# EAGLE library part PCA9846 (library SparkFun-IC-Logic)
NXP Semiconductors PCA9846 - I2C Multiplexer The PCA9846 device has four bidirectional translating switches that can be controlled through the I2C bus. The SCL/SDA upstream pair fans out to four downstream pairs, or channels. Any individual SCn/SDn channel or combination of channels can be selected, determined by the contents of the programmable control register. These downstream channels can be used to resolve I2C address conflicts.
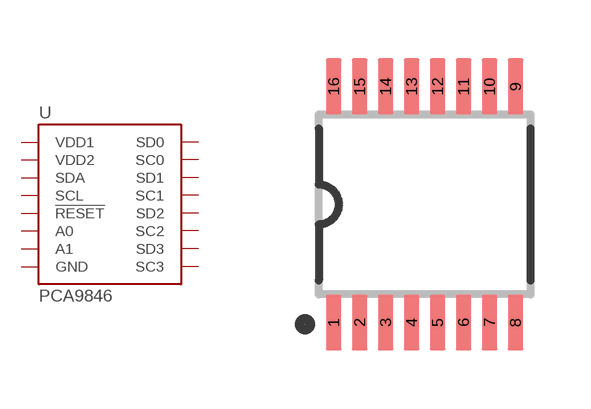
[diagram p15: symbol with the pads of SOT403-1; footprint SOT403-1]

Designator prefix U

## PCA9846 (PROD_ID: IC-18372)  [SOT403-1]
1  VDD1  pwr
2  A0
3  !RESET  in
4  SD0
5  SC0
6  SD1
7  SC1
8  GND  pwr
9  SD2
10  SC2
11  SD3
12  SC3
13  A1
14  SCL
15  SDA
16  VDD2  pwr

## Footprint SOT403-1 (pad centres in mm)
SOT403-1 TSSOP16 thin small outline package
smd 0.4 x 1.4: 1 -2.275,-2.95; 2 -1.625,-2.95; 3 -0.975,-2.95; 4 -0.325,-2.95; 5 0.325,-2.95; 6 0.975,-2.95; 7 1.625,-2.95; 8 2.275,-2.95; 9 2.275,2.95; 10 1.625,2.95; 11 0.975,2.95; 12 0.325,2.95; 13 -0.325,2.95; 14 -0.975,2.95; 15 -1.625,2.95; 16 -2.275,2.95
